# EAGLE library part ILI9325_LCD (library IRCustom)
2.8" ILI9325-based TFT LCD w/Integrated Touch Screen
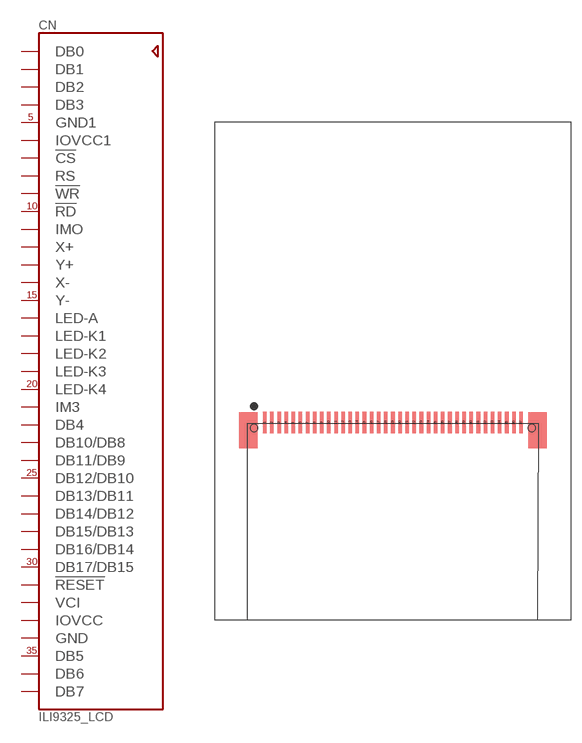
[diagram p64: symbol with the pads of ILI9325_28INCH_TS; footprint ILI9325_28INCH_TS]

Designator prefix CN

## ILI9325_LCD1.0MM  [ILI9325_28INCH_TS]
1  DB0  pas
2  DB1  pas
3  DB2  pas
4  DB3  pas
5  GND1  pwr
6  IOVCC1  pwr
7  !CS  pas
8  RS  pas
9  !WR  pas
10  !RD  pas
11  IMO  pas
12  X+  pas
13  Y+  pas
14  X-  pas
15  Y-  pas
16  LED-A  pas
17  LED-K1  pas
18  LED-K2  pas
19  LED-K3  pas
20  LED-K4  pas
21  IM3  pas
22  DB4  pas
23  DB10/DB8  pas
24  DB11/DB9  pas
25  DB12/DB10  pas
26  DB13/DB11  pas
27  DB14/DB12  pas
28  DB15/DB13  pas
29  DB16/DB14  pas
30  DB17/DB15  pas
31  !RESET  pas
32  VCI  pwr
33  IOVCC  pwr
34  GND  pwr
35  DB5  pas
36  DB6  pas
37  DB7  pas

## Footprint ILI9325_28INCH_TS (pad centres in mm)
1.0mm-Pitch 37 Pin LCD Connector
smd 0.5 x 3: 1 -18,27.77; 2 -17,27.77; 3 -16,27.77; 4 -15,27.77; 5 -14,27.77; 6 -13,27.77; 7 -12,27.77; 8 -11,27.77; 9 -10,27.77; 10 -9,27.77; 11 -8,27.77; 12 -7,27.77; 13 -6,27.77; 14 -5,27.77; 15 -4,27.77; 16 -3,27.77; 17 -2,27.77; 18 -1,27.77; 19 0,27.77; 20 1,27.77; 21 2,27.77; 22 3,27.77; 23 4,27.77; 24 5,27.77; 25 6,27.77; 26 7,27.77; 27 8,27.77; 28 9,27.77; 29 10,27.77; 30 11,27.77; 31 12,27.77; 32 13,27.77; 33 14,27.77; 34 15,27.77; 35 16,27.77; 36 17,27.77; 37 18,27.77
hole 1 at -19.5,27
hole 1 at 19.5,27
